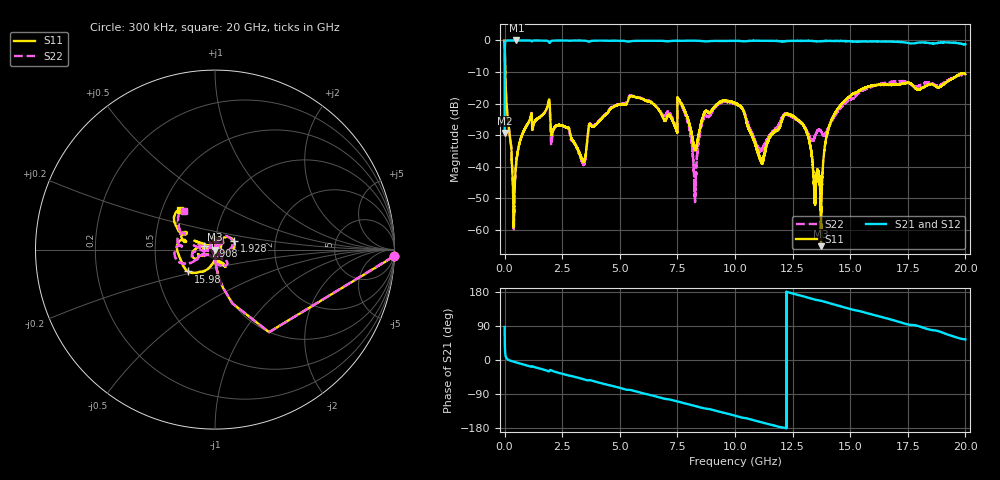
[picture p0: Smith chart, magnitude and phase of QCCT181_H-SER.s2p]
! Created Fri Feb  5 15:35:09 2021
# hz S ma R 50
! 2 Port Network Data from SP1.SP block
! freq  magS11  angS11  magS21  angS21  magS12  angS12  magS22  angS22
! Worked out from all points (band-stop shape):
!   20001 points, 300 kHz to 20 GHz, reference 50 ohm
!   highest |S21| = -0.01 dB at 510.3 MHz (marker M1); lowest = -29.3 dB at 300 kHz (marker M2)
!   |S21| within 3 dB of the highest: 8.824 MHz to end of sweep
!   lowest |S11| = -65.2 dB at 13.73 GHz (marker M3), VSWR 1.00, Z = 50 - j0.0266 ohm
!   |S11| at or under -10 dB: 26.19 MHz to end of sweep
!   |S22| runs from -60.4 to 0.0 dB; largest |S21 - S12| = 0.014
!   S11 on the Smith chart (normalised r, x): 300 kHz: 3, -52; 1.928 GHz: 1.23, +0.12; 7.908 GHz: 0.89, +0.03; 15.98 GHz: 0.72, -0.18; 20 GHz: 0.62, +0.30
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300000  0.9982 -2.2  0.0341 87.3  0.03434 87.9  0.9955 -2.1
1.043e8  0.08021 -87.3  0.996 3.2  0.996 3.3  0.08055 -87.2
3.483e8  0.006522 -104.6  0.9988 -3.7  0.9987 -3.6  0.006771 -104.0
5.103e8  0.01194 89.2  0.9994 -6.6  0.9975 -6.6  0.01186 88.5
1.0813e9  0.05415 73.2  0.9966 -16.0  0.9971 -16.0  0.0538 74.4
1.9283e9  0.1161 23.8  0.9321 -30.2  0.9312 -30.2  0.1077 28.9
3.3343e9  0.0138 22.5  0.995 -49.2  0.9952 -49.2  0.0127 42.9
3.7143e9  0.0472 -108.8  0.9695 -53.3  0.9693 -53.2  0.04812 -111.0
4.6623e9  0.08629 -158.5  0.9889 -68.2  0.9891 -68.2  0.08874 -153.8
6.6673e9  0.08197 169.0  0.9878 -97.8  0.9877 -97.8  0.08322 -178.4
7.9083e9  0.06274 162.6  0.9885 -115.8  0.9888 -115.8  0.0575 163.5
8.2653e9  0.01897 -136.5  0.9892 -121.3  0.9885 -121.3  0.003393 -119.7
8.6603e9  0.07032 -70.4  0.9723 -127.5  0.9732 -127.5  0.06122 -49.3
1.00003e10  0.1015 -59.5  0.9847 -146.9  0.9859 -147.0  0.09919 -64.2
1.11323e10  0.01247 9.9  0.9865 -164.2  0.9874 -164.1  0.01885 -167.5
1.22443e10  0.06782 88.4  0.9784 179.6  0.9771 179.7  0.06719 105.7
1.33343e10  0.01524 62.3  0.9831 161.7  0.9828 161.6  0.02626 119.3
1.37333e10  0.0005506 -151.1  0.9697 156.3  0.9696 156.3  0.03641 146.7
1.42653e10  0.06223 -94.6  0.9838 147.1  0.9837 147.1  0.05824 -162.2
1.59833e10  0.1925 -140.9  0.9636 119.5  0.9646 119.5  0.1882 -155.5
1.66673e10  0.1974 -156.2  0.9585 108.4  0.9509 108.3  0.2163 -162.3
2e10  0.2923 131.7  0.8672 54.5  0.8596 54.2  0.2769 128.8
